(* Logix 5000 AddOnInstructionDefinition export ACS_INCREMENTAL_ROTARY_MOVE; software revision 24.00 *)

ADD_ON_INSTRUCTION ACS_INCREMENTAL_ROTARY_MOVE   (* revision 1.0, vendor Tolomatic, Inc. *)
VAR_INPUT
   Distance : REAL; {required}   // Distance to Travel (Positive or Negative)
   Acceleration : REAL; {required}   // Trajectory Acceleration
   Deceleration : REAL; {required}   // Trajectory Deceleration
   Velocity : REAL; {required}   // Trajectory Constance Velocity
   Force : REAL; {required}   // Force Limit (Percent)
END_VAR
VAR_IN_OUT
   DriveMoveSelect : SINT; {required}   // ACS.O.MOVESELECT
   DriveTargetAcc : REAL; {required}   // ACS.O.TARGET_0_ACC
   DriveTargetDec : REAL; {required}   // ACS.O.TARGET_0_DEC
   DriveTargetForce : REAL; {required}   // ACS.O.TARGET_0_FORCE
   DriveTargetMotionType : DINT; {required}   // ACS.O.TARGET_0_MOTION_TYPE
   DriveTargetPos : REAL; {required}   // ACS.O.TARGET_0_POS
   DriveTargetVel : REAL; {required}   // ACS.O.TARGET_0_VEL
END_VAR
VAR
   AbsDistance : REAL; {access None}   // Absolute Value of Distance Input
END_VAR

ROUTINE Logic   (* ladder *)
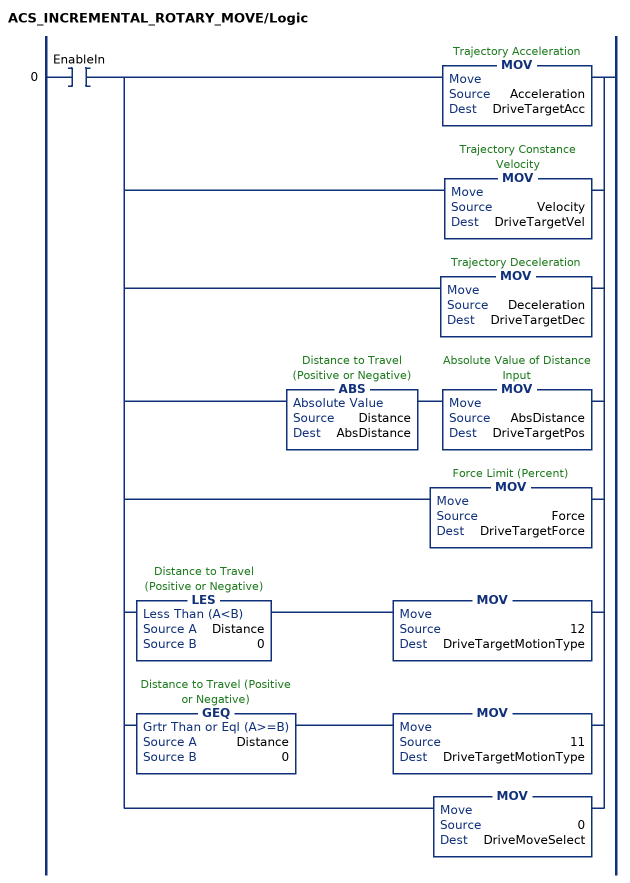
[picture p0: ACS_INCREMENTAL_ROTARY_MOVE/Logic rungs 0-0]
   0: XIC(EnableIn)[MOV(Acceleration,DriveTargetAcc) ,MOV(Velocity,DriveTargetVel) ,MOV(Deceleration,DriveTargetDec) ,ABS(Distance,AbsDistance) MOV(AbsDistance,DriveTargetPos) ,MOV(Force,DriveTargetForce) ,LES(Distance,0) MOV(12,DriveTargetMotionType) ,GEQ(Distance,0) MOV(11,DriveTargetMotionType) ,MOV(0,DriveMoveSelect) ];
END_ROUTINE
END_ADD_ON_INSTRUCTION
